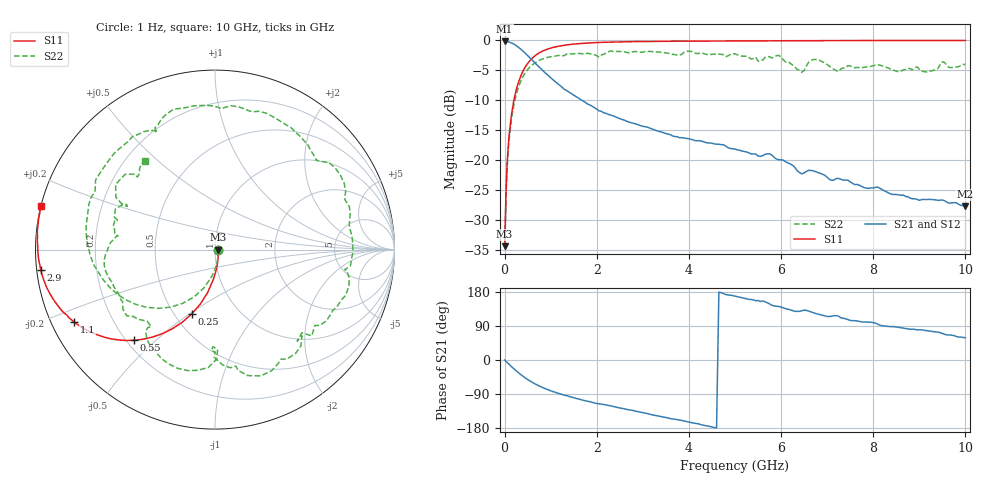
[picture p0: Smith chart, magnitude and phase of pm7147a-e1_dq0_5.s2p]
# GHz S DB R 50
! S-Parameters data
! Freq  dbS11  angS11  dbS21  angS21  dbS12  angS12  dbS22  angS22
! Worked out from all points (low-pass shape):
!   279 points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, 1 Hz to 10 GHz, reference 50 ohm
!   highest |S21| = -0.17 dB at 1.259 kHz (marker M1); lowest = -27.8 dB at 10 GHz (marker M2)
!   |S21| within 3 dB of the highest: start of sweep to 581.5 MHz
!   lowest |S11| = -34.4 dB at 794.3 Hz (marker M3), VSWR 1.04, Z = 51.9 - j0.000132 ohm
!   |S11| at or under -10 dB: start of sweep to 201.9 MHz
!   |S22| runs from -34.4 to -1.8 dB; largest |S21 - S12| = 2.6e-13
!   S11 on the Smith chart (normalised r, x): 1 Hz: 1.04, -0.00; 250 MHz: 0.61, -0.51; 550 MHz: 0.23, -0.43; 1.1 GHz: 0.07, -0.24; 2.9 GHz: 0.01, -0.06; 10 GHz: 0.00, +0.12
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1e-09  -34.44 -0.0  -0.17 -0.0  -0.17 -0.0  -34.44 -0.0
7.943e-07  -34.44 -0.0  -0.17 -0.0  -0.17 -0.0  -34.44 -0.0
1.2589e-06  -34.44 -0.0  -0.17 -0.0  -0.17 -0.0  -34.44 -0.0
0.03981072  -23.34 -77.3  -0.19 -4.7  -0.19 -4.7  -24.00 -77.8
0.07943282  -17.65 -89.3  -0.24 -9.4  -0.24 -9.4  -18.34 -92.2
0.25  -8.35 -109.9  -0.87 -28.5  -0.87 -28.5  -9.13 -121.0
0.55  -3.38 -131.8  -2.92 -55.4  -2.92 -55.4  -4.45 -155.7
1.1  -1.09 -152.8  -6.92 -85.3  -6.92 -85.3  -2.63 163.6
1.7  -0.49 -163.4  -10.13 -106.0  -10.13 -106.0  -2.23 131.1
2.3  -0.29 -169.4  -12.49 -120.9  -12.49 -120.9  -1.77 106.5
2.9  -0.20 -173.5  -14.13 -136.5  -14.13 -136.5  -1.93 78.2
3.35  -0.16 -175.7  -15.22 -148.1  -15.22 -148.1  -1.94 57.8
4.1  -0.11 -178.9  -16.69 -166.5  -16.69 -166.5  -1.97 23.9
5.05  -0.09 177.9  -18.32 167.1  -18.32 167.1  -2.42 -21.9
5.95  -0.07 175.4  -19.97 141.2  -19.97 141.2  -2.52 -70.1
6.45  -0.04 174.0  -22.35 130.1  -22.35 130.1  -5.33 -91.1
6.7  -0.04 173.4  -21.83 124.7  -21.83 124.7  -3.21 -102.7
6.95  -0.04 172.7  -22.58 116.4  -22.58 116.4  -3.77 -123.6
7.5  -0.03 171.4  -23.67 104.4  -23.67 104.4  -4.28 -147.1
8.35  -0.02 169.4  -25.60 88.3  -25.60 88.3  -4.70 176.0
9.5  -0.01 166.8  -26.71 70.0  -26.71 70.0  -3.58 146.7
10  -0.01 165.8  -27.78 58.8  -27.78 58.8  -4.05 128.3
